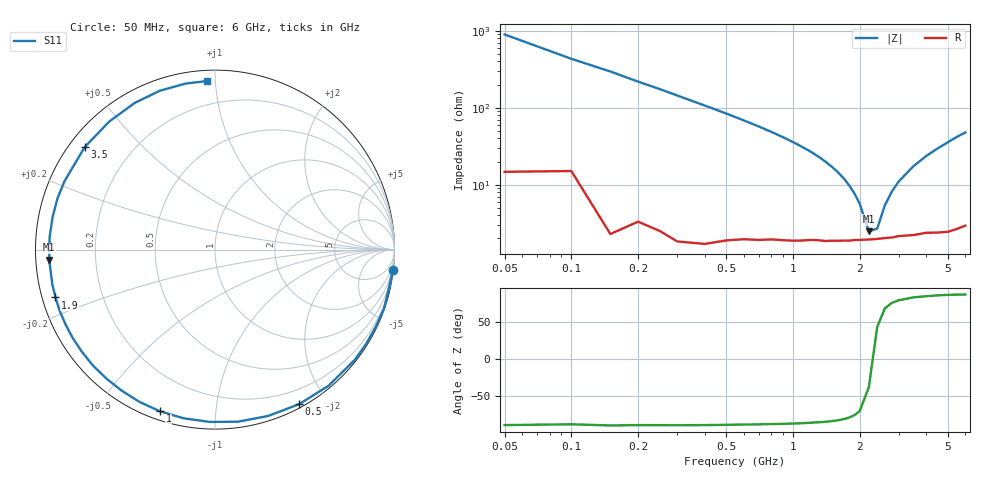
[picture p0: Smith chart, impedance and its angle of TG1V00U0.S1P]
! SIEMENS Discrete & RF Semiconductors
! BAT64
! Si Schottky Diode in SOT23
! VR = 1 V
! S-Parameters:  February  1997
# GHz  S  MA  R  50
!  f  S11
! GHz  MAG  ANG
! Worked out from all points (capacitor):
!   34 points, 50 MHz to 6 GHz, reference 50 ohm
!   read as one part to ground: C = 3.57 pF near 50 MHz
!   lowest |Z| = 2.47 ohm at 2.2 GHz (marker M1)
!   series resonance near 2.291 GHz, so ESL is about 1.4 nH
!   S11 on the Smith chart (normalised r, x): 50 MHz: 0, -18; 500 MHz: 0.04, -1.68; 1 GHz: 0.04, -0.72; 1.9 GHz: 0.04, -0.15; 3.5 GHz: 0.04, +0.35; 6 GHz: 0.06, +0.95
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0.05  0.9982 -6.4
0.1  0.9921 -13.2
0.15  0.9975 -19.2
0.2  0.9934 -25.8
0.3  0.9922 -38.2
0.4  0.9878 -50.2
0.5  0.9805 -61.5
0.6  0.9731 -72.3
0.7  0.9673 -82.4
0.8  0.9607 -91.8
0.9  0.9559 -100.6
1  0.9516 -108.8
1.1  0.947 -116.4
1.3  0.9393 -130.2
1.4  0.938 -136.6
1.6  0.9332 -148.1
1.8  0.93 -158.5
1.9  0.9278 -163.3
2.2  0.9253 -176.5
2.4  0.9243 175.8
2.6  0.9228 168.5
3  0.9211 155.6
3.5  0.9238 141.8
4  0.9252 129.5
4.5  0.9316 118.8
5  0.937 109.2
5.5  0.9392 100.1
6  0.9403 92.7
